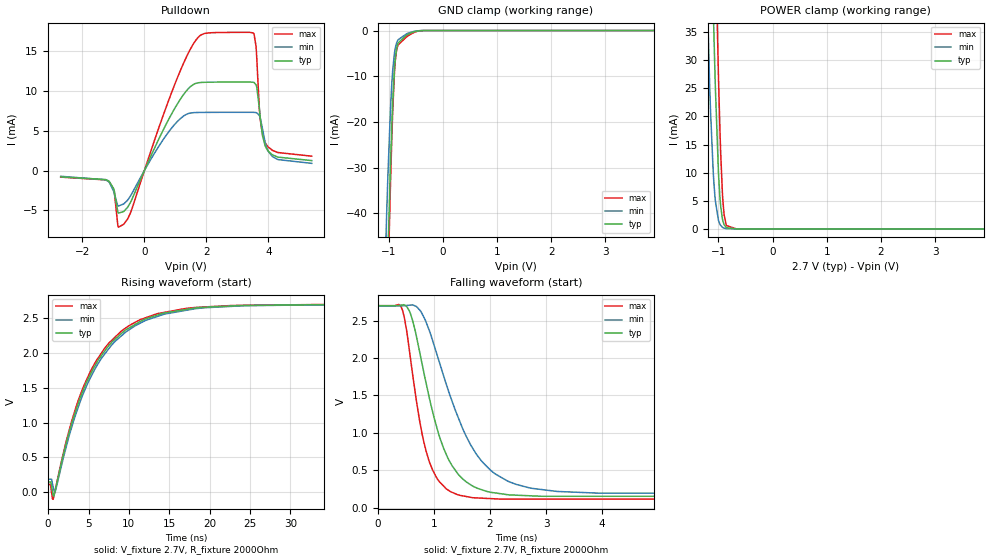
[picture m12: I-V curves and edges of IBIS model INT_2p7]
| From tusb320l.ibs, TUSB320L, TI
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|   Model
[Model]   INT_2p7
Model_type   Open_drain
Polarity   Non-Inverting
Vmeas = 1.35
Vref = 2.7
Cref = 1pF
Rref = 2000
|   typ   min   max
C_comp   0.595pF   0.579pF   0.649pF
[Voltage Range]   2.7   2.699   2.701
[Temperature Range]   27   105   -40
[Pullup Reference]   2.7   2.699   2.701
[Pulldown Reference]   0   0   -0
[Power Clamp Reference]   2.7   2.699   2.701
[GND Clamp Reference]   0   0   0
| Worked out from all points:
|   slope of the pulldown table from 0 to 0.405 V, typ, clamps not added: 117 ohm
|   GND clamp passes 1 mA (typ) near -0.67 V on its own axis
|   POWER clamp passes 1 mA (typ) near -0.90 V on its own axis
|   falling waveform, V_fixture 2.7V, R_fixture 2000Ohm: 20-80 % time 537ps typ, 789ps min, 364ps max; typ from 2.7 V to 0.146 V
|   rising waveform, V_fixture 2.7V, R_fixture 2000Ohm: 20-80 % time 6.03ns typ, 6.23ns min, 5.84ns max; typ from 0.146 V to 2.7 V
[Pulldown]
|   Voltage   I(typ)   I(min)   I(max)
-2.7V     -790.2uA   -720.5uA   -826.2uA
-1.137V   -1.353mA   -1.451mA   -1.397mA
-966.6mV  -2.636mA   -2.992mA   -2.842mA
-845.1mV  -5.282mA   -4.44mA    -7.024mA
-666.9mV  -5.137mA   -4.186mA   -6.741mA
1.147V    8.871mA    6.467mA    12.42mA
2.055V    11.08mA    7.295mA    17.25mA
3.521V    11.06mA    7.297mA    17.22mA
3.602V    10.75mA    7.264mA    15.57mA
3.74V     6.505mA    6.568mA    6.324mA
3.893V    3.135mA    3.565mA    3.536mA
5.4V      1.246mA    899.4uA    1.8mA
[GND Clamp]
|   Voltage   I(typ)   I(min)   I(max)
-2.7V     -998.5mA   -936.5mA   -1.04A
-1.056V   -68.01mA   -47.43mA   -76.49mA
-1.04V    -60.34mA   -40.99mA   -68.16mA
-1.015V   -49.25mA   -31.98mA   -55.99mA
-966.6mV  -29.14mA   -17.04mA   -33.4mA
-942.3mV  -20.64mA   -11.56mA   -23.54mA
-893.7mV  -8.522mA   -4.951mA   -9.148mA
-877.5mV  -6.151mA   -3.8mA     -6.462mA
-828.9mV  -2.767mA   -2.052mA   -3.183mA
-666.9mV  -968.4uA   -702.9uA   -1.36mA
-351mV    -7.091uA   -6.604uA   -8.492uA
5.4V      0A         0A         0A
[POWER Clamp]
|   Voltage   I(typ)   I(min)   I(max)
-2.7V     943.9mA    860.1mA    1.001A
-1.242V   107.3mA    54.31mA    147.1mA
-1.161V   67.86mA    25.44mA    103.6mA
-1.088V   36.66mA    8.959mA    66.56mA
-1.056V   25.04mA    4.964mA    51.17mA
-999mV    9.991mA    1.542mA    27.12mA
-958.5mV  4.108mA    631uA      13.69mA
-926.1mV  1.8mA      304.1uA    6.411mA
-893.7mV  742.9uA    145.6uA    2.45mA
-853.2mV  236.4uA    57.74uA    608.8uA
-666.9mV  1.096uA    801.7nA    615.8nA
5.4V      0A         0A         0A
[Ramp]
R_load = 2000
|   typ   min   max
dV/dt_r   1.53224/6.00713e-09   1.50834/6.21935e-09   1.55462/5.79984e-09
dV/dt_f   1.53224/5.3523e-10   1.50834/7.86905e-10   1.55462/3.62888e-10
[Falling Waveform]
V_fixture = 2.7V
V_fixture_min = 2.699V
V_fixture_max = 2.701V
R_fixture = 2000Ohm
C_fixture = 0F
|   Time   V(typ)   V(min)   V(max)
0s        2.7V       2.699V     2.701V
433.3ps   2.71V      2.699V     2.654V
584.9ps   2.585V     2.709V     1.975V
787.2ps   1.926V     2.595V     990.4mV
1.048ns   1.078V     2.061V     397.9mV
1.322ns   560.9mV    1.424V     204mV
1.652ns   305.6mV    841.2mV    136.8mV
2.189ns   185.1mV    408.1mV    113mV
3.951ns   150.9mV    192.2mV    113mV
200ns     146.3mV    185.1mV    110mV
[Rising Waveform]
V_fixture = 2.7V
V_fixture_min = 2.699V
V_fixture_max = 2.701V
R_fixture = 2000Ohm
C_fixture = 0F
|   Time   V(typ)   V(min)   V(max)
0s        146.3mV    185.1mV    110mV
281.4ps   145.9mV    184.8mV    109.2mV
536ps     8.179mV    119.3mV    -98.75mV
876.3ps   25.29mV    10.54mV    31.25mV
2.276ns   719.3mV    668.6mV    749.9mV
3.771ns   1.293V     1.236V     1.332V
6.982ns   2.027V     1.984V     2.068V
10.71ns   2.409V     2.39V      2.44V
17.11ns   2.63V      2.618V     2.645V
200ns     2.7V       2.699V     2.701V
